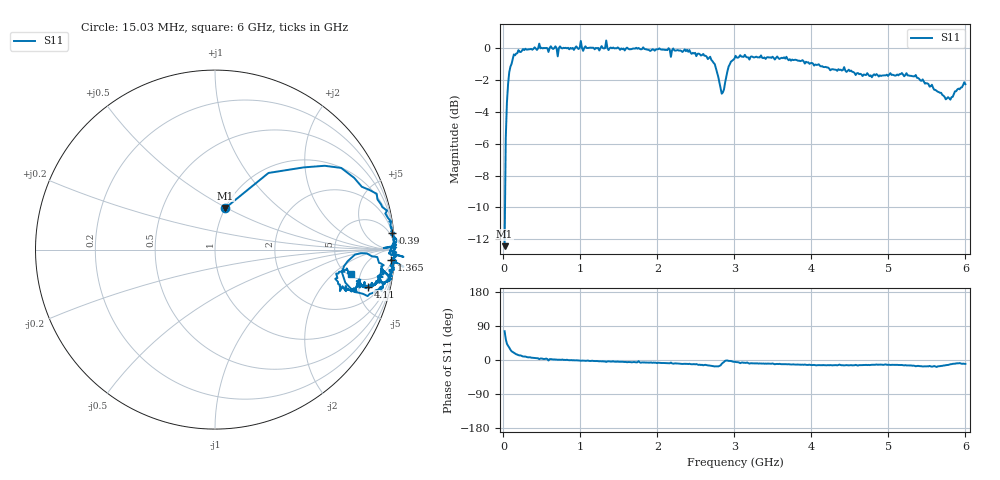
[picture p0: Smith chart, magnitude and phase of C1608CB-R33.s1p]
!	Network	Analyzer	HP8753E.07.74:	Oct	30	2002	Serial	No.	JP38451487
!	Hewlett-Packard
!	28	Aug	2009	8:44:22
!	Frequency	S11
#	HZ	S	RI	R	50
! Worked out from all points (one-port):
!   400 points, 15.03 MHz to 6 GHz, reference 50 ohm
!   lowest |S11| = -12.4 dB at 15.03 MHz (marker M1), VSWR 1.63, Z = 50.1 + j24.6 ohm
!   |S11| at or under -10 dB: start of sweep to 20.42 MHz
!   S11 on the Smith chart (normalised r, x): 15.03 MHz: 1.00, +0.49; 390 MHz: 2, +21; 1.365 GHz: 8, -31; 4.11 GHz: 3.52, -6.44; 6 GHz: 5.27, -3.51
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1.502992e7  0.058 0.232
3.002985e7  0.298 0.427
4.502978e7  0.494 0.458
9.002955e7  0.775 0.4
1.350293e8  0.901 0.311
3.90028e8  0.988 0.0949
5.550272e8  0.997 0.0654
5.850271e8  0.97 -0.0229
7.650262e8  0.995 0.0211
1.005025e9  1.05 -0.0403
1.035025e9  0.978 -0.0274
1.245024e9  0.979 -0.0595
1.335023e9  1.05 -0.0955
1.365023e9  0.982 -0.0598
1.515022e9  0.982 -0.0794
2.265019e9  0.971 -0.158
2.685017e9  0.906 -0.241
2.790016e9  0.776 -0.236
2.835016e9  0.707 -0.126
2.895016e9  0.813 -0.0202
3.015015e9  0.94 -0.0869
3.765011e9  0.897 -0.181
4.110009e9  0.854 -0.208
4.515007e9  0.825 -0.199
5.265004e9  0.793 -0.205
5.625002e9  0.696 -0.231
5.745001e9  0.67 -0.163
6e9  0.757 -0.136
